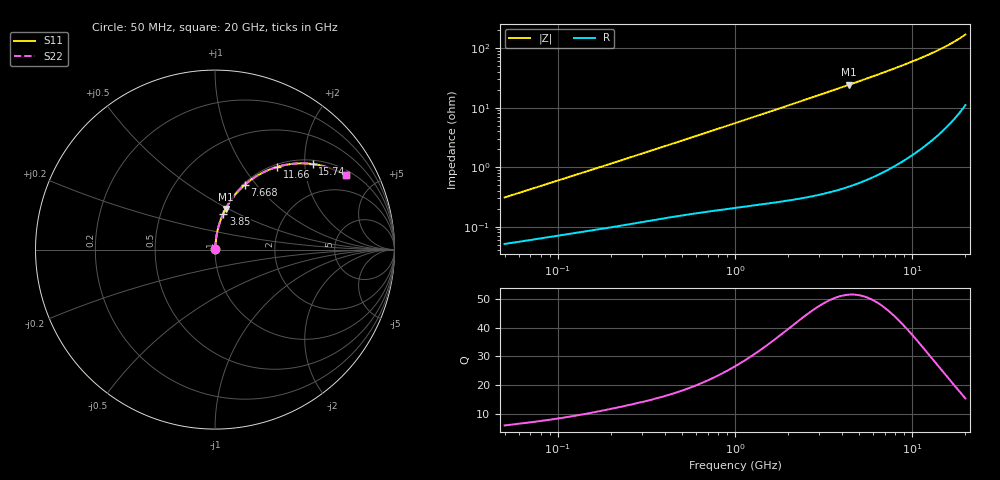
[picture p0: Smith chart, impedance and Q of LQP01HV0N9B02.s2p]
!Murata Part Number: LQP01HV0N9B02
!These Parameters are Measured in Series Mode Connection
!  o--[Z]--o
!Port1  Port2
!  o-------o
!Freq. Start=50[MHz] Stop=20[GHz], 401[Steps]
# Hz S RI R 50
!Freq.(Hz) S11(Real) S11(Imag) S21(Real) S21(Imag) S12(Real) S12(Imag) S22(Real) S22(Imag)
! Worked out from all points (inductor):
!   401 points, 50 MHz to 20 GHz, reference 50 ohm
!   read as one part in series: L = 961 pH near 51.52 MHz
!   highest Q = 51.5 at 4.406 GHz (marker M1), where L = 876 pH
!   S11 on the Smith chart (normalised r, x): 50 MHz: 1.00, +0.01; 3.85 GHz: 1.01, +0.42; 7.668 GHz: 1.02, +0.87; 11.66 GHz: 1.04, +1.44; 15.74 GHz: 1.10, +2.19; 20 GHz: 1.22, +3.39
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5e7  0.000522 0.00305  0.9995 -0.00305  0.9995 -0.00305  0.000522 0.00305
5.152053e7  0.00053 0.00314  0.9995 -0.00314  0.9995 -0.00314  0.00053 0.00314
1.364002e8  0.000877 0.00793  0.9991 -0.00793  0.9991 -0.00793  0.000877 0.00793
3.721004e8  0.00177 0.0208  0.9982 -0.0208  0.9982 -0.0208  0.00177 0.0208
6.380365e8  0.00295 0.0351  0.9971 -0.0351  0.9971 -0.0351  0.00295 0.0351
1e9  0.00503 0.0544  0.995 -0.0544  0.995 -0.0544  0.00503 0.0544
1.714689e9  0.0111 0.0921  0.9889 -0.0921  0.9889 -0.0921  0.0111 0.0921
2.728004e9  0.0247 0.1446  0.9753 -0.1446  0.9753 -0.1446  0.0247 0.1446
3.850025e9  0.0462 0.2004  0.9538 -0.2004  0.9538 -0.2004  0.0462 0.2004
4.405649e9  0.0594 0.2269  0.9406 -0.2269  0.9406 -0.2269  0.0594 0.2269
5.856089e9  0.1011 0.2916  0.8989 -0.2916  0.8989 -0.2916  0.1011 0.2916
7.442007e9  0.1573 0.3533  0.8427 -0.3533  0.8427 -0.3533  0.1573 0.3533
7.668323e9  0.1661 0.3612  0.8339 -0.3612  0.8339 -0.3612  0.1661 0.3612
8.516016e9  0.2007 0.3889  0.7993 -0.3889  0.7993 -0.3889  0.2007 0.3889
9.457416e9  0.2417 0.4155  0.7583 -0.4155  0.7583 -0.4155  0.2417 0.4155
1.050288e10  0.2896 0.4399  0.7104 -0.4399  0.7104 -0.4399  0.2896 0.4399
1.166392e10  0.3451 0.4604  0.6549 -0.4604  0.6549 -0.4604  0.3451 0.4604
1.375312e10  0.4477 0.4793  0.5523 -0.4793  0.5523 -0.4793  0.4477 0.4793
1.573793e10  0.5441 0.4768  0.4559 -0.4768  0.4559 -0.4768  0.5441 0.4768
1.747767e10  0.6245 0.4594  0.3755 -0.4594  0.3755 -0.4594  0.6245 0.4594
1.940974e10  0.7062 0.4259  0.2938 -0.4259  0.2938 -0.4259  0.7062 0.4259
2e10  0.7292 0.413  0.2708 -0.413  0.2708 -0.413  0.7292 0.413
